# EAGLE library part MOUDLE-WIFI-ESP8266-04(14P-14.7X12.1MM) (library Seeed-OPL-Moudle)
114990085
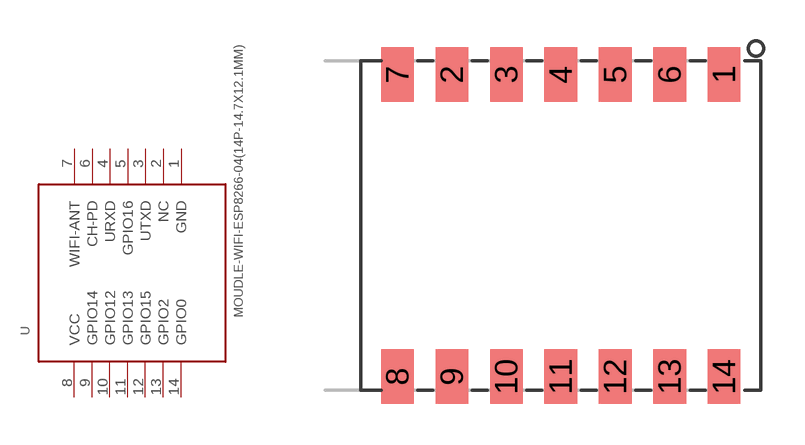
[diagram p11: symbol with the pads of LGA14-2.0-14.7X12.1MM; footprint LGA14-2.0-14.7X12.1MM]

Designator prefix U

## MOUDLE-WIFI-ESP8266-04(14P-14.7X12.1MM) (MPN: ESP8266-04; VALUE: ESP8266-04)  [LGA14-2.0-14.7X12.1MM]
1  GND
2  NC
3  UTXD
4  URXD
5  GPIO16
6  CH-PD
7  WIFI-ANT
8  VCC
9  GPIO14
10  GPIO12
11  GPIO13
12  GPIO15
13  GPIO2
14  GPIO0

## Footprint LGA14-2.0-14.7X12.1MM (pad centres in mm)
smd 1.2 x 2: 1 6,5.55; 2 -4,5.55; 3 -2,5.55; 4 0,5.55; 5 2,5.55; 6 4,5.55; 7 -6,5.55; 8 -6,-5.55; 9 -4,-5.55; 10 -2,-5.55; 11 0,-5.55; 12 2,-5.55; 13 4,-5.55; 14 6,-5.55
